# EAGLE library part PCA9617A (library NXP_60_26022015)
Level translating Fm+ I2C-bus repeater The PCA9617A is a CMOS integrated circuit that provides level shifting between low voltage (0.8 V to 5.5 V) and higher voltage (2.2 V to 5.5 V) Fast-mode Plus (Fm+) I2 C-bus or SMBus applications. While retaining all the operating modes and features of the I 2 C-bus system during the level shifts, it also permits extension of the I2 C-bus by providing bidirectional buffering for both the data (SDA) and the clock (SCL) lines, thus enabling two buses of 540 pF at 1 MHz or up to 4000 pF at lower speeds. Using the PCA9617A enables the system designer to isolate two halves of a bus for both voltage and capacitance. The SDA and SCL pins are overvoltage tolerant and are high-impedance when the PCA9617A is unpowered. The 2.2 V to 5.5 V bus port B drivers have the static level offset, while the adjustable voltage bus port A drivers eliminate the static offset voltage. This results in a LOW on the port B translating into a nearly 0 V LOW on the port A which accommodates the smaller voltage swings of lower voltage logic. The static offset design of the port B PCA9617A I/O drivers prevents them from being connected to the static or incremented offset of other bus buffers. Port A of two or more PCA9617As can be connected together, however, to allow a star topography with port A on the common bus, and port A can be connected directly to any other buffer with static or incremented offset outputs. Multiple PCA9617As can be connected in series, port A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
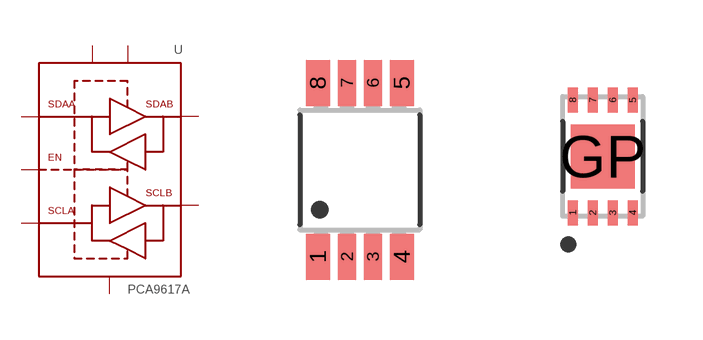
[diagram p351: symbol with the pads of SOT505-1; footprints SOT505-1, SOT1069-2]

Designator prefix U

## PCA9617ADP  [SOT505-1]
1  VCC(A)  pwr
2  SCLA
3  SDAA
4  GND  pwr
5  EN  in
6  SDAB
7  SCLB
8  VCC(B)  pwr

## PCA9617ATP  [SOT1069-2]
1  SDAA
2  GND  pwr
3  EN  in
4  SDAB
5  SCLB
6  VCC(B)  pwr
7  VCC(A)  pwr
8  SCLA

## Footprint SOT505-1 (pad centres in mm)
SOT505-1 TSSOP8: plastic thin shrink small outline package; 8 leads; body width 3 mm JEDEC: -- IEC: --
smd 0.6 x 1.15: 1 -1.05,-2.175; 4 1.05,-2.175; 5 1.05,2.175; 8 -1.05,2.175
smd 0.45 x 1.15: 2 -0.325,-2.175; 3 0.325,-2.175; 6 0.325,2.175; 7 -0.325,2.175

## Footprint SOT1069-2 (pad centres in mm)
SOT1069 HWSON8: plastic thermal enhanced very very thin small outline package; no leads;8 terminals; body 2 x 3 x 0.75 mm JEDEC: IEC: -- JEITA: --
smd 0.25 x 0.625: 1 -0.75,-1.413; 2 -0.25,-1.413; 3 0.25,-1.413; 4 0.75,-1.413; 5 0.75,1.413; 6 0.25,1.413; 7 -0.25,1.413; 8 -0.75,1.413
smd 1.6 x 1.6: GP 0,0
